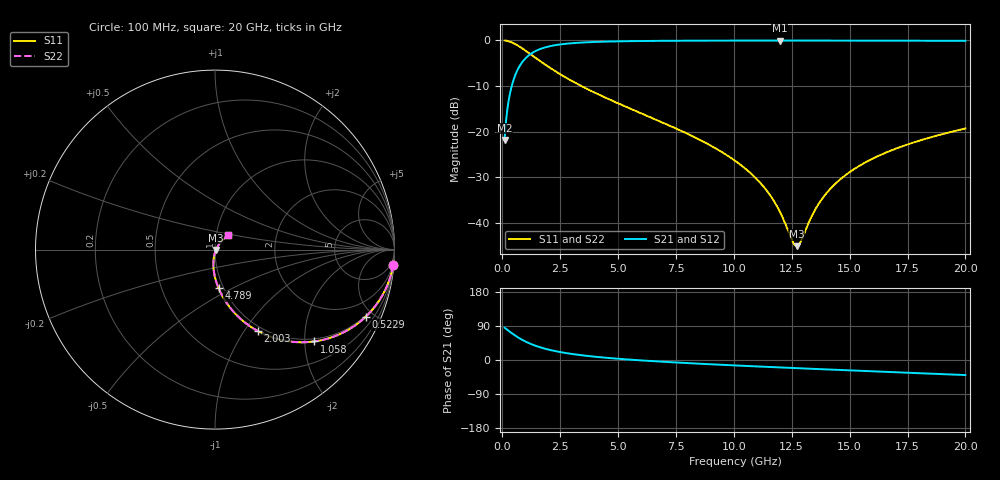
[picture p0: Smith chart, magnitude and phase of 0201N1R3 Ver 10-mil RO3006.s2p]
# GHz S MA R 50
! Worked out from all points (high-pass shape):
!   1601 points, 100 MHz to 20 GHz, reference 50 ohm
!   highest |S21| = -0.05 dB at 11.98 GHz (marker M1); lowest = -21.8 dB at 100 MHz (marker M2)
!   |S21| within 3 dB of the highest: 1.206 GHz to end of sweep
!   lowest |S11| = -45.0 dB at 12.71 GHz (marker M3), VSWR 1.01, Z = 50.5 - j0.212 ohm
!   |S11| at or under -10 dB: 3.416 GHz to end of sweep
!   |S22| runs from -45.0 to 0.0 dB; largest |S21 - S12| = 0
!   S11 on the Smith chart (normalised r, x): 100 MHz: 1, -24; 522.9 MHz: 0.94, -4.51; 1.058 GHz: 0.94, -2.22; 2.003 GHz: 0.94, -1.15; 4.789 GHz: 0.95, -0.43; 20 GHz: 1.15, +0.18
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0.1  0.9967 -4.8  0.08145 85.1  0.08145 85.1  0.9967 -4.8
0.299  0.9713 -14.2  0.2374 75.7  0.2374 75.7  0.9713 -14.2
0.522875  0.919 -24.1  0.3933 65.9  0.3933 65.9  0.919 -24.1
0.7591875  0.8484 -33.2  0.528 56.7  0.528 56.7  0.8484 -33.2
1.057687  0.7536 -42.8  0.6555 47.1  0.6555 47.1  0.7536 -42.8
1.505437  0.6248 -53.7  0.7785 36.1  0.7785 36.1  0.6248 -53.7
2.002937  0.5115 -62.4  0.8566 27.3  0.8566 27.3  0.5115 -62.4
3.420812  0.3158 -76.8  0.9454 12.6  0.9454 12.6  0.3158 -76.8
4.788938  0.216 -84.7  0.9724 4.3  0.9724 4.3  0.216 -84.7
6.741625  0.1321 -92.0  0.9867 -3.9  0.9867 -3.9  0.1321 -92.0
8.694313  0.07759 -96.8  0.992 -10.4  0.992 -10.4  0.07759 -96.8
10.05  0.04818 -98.3  0.9935 -14.3  0.9935 -14.3  0.04818 -98.3
11.18181  0.02687 -96.1  0.9941 -17.5  0.9941 -17.5  0.02687 -96.1
11.97781  0.01348 -85.7  0.9942 -19.6  0.9942 -19.6  0.01348 -85.7
12.52506  0.006373 -50.3  0.9941 -21.1  0.9941 -21.1  0.006373 -50.3
12.71162  0.005593 -22.0  0.9941 -21.5  0.9941 -21.5  0.005593 -22.0
12.88575  0.006281 4.4  0.994 -22.0  0.994 -22.0  0.006281 4.4
13.37081  0.01202 38.4  0.9939 -23.2  0.9939 -23.2  0.01202 38.4
13.91806  0.02002 48.5  0.9937 -24.6  0.9937 -24.6  0.02002 48.5
14.61456  0.03041 52.3  0.9932 -26.4  0.9932 -26.4  0.03041 52.3
16.69162  0.06085 52.5  0.9914 -31.6  0.9914 -31.6  0.06085 52.5
20  0.1084 46.6  0.9867 -39.7  0.9867 -39.7  0.1084 46.6
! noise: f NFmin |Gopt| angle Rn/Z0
0.1  0.0009838  0.9589  0.8362  0.005397
2.301  0.005361  0.8263  4.478  0.006477
4.515  0.008286  0.7844  8.121  0.007859
6.729  0.01081  0.7578  11.78  0.008935
8.943  0.01311  0.7382  15.41  0.009849
11.14  0.01527  0.7232  19.01  0.01065
13.36  0.01735  0.7111  22.58  0.01139
15.57  0.01936  0.7014  26.12  0.01207
17.79  0.02134  0.6935  29.62  0.01272
20  0.02329  0.6872  33.07  0.01333
